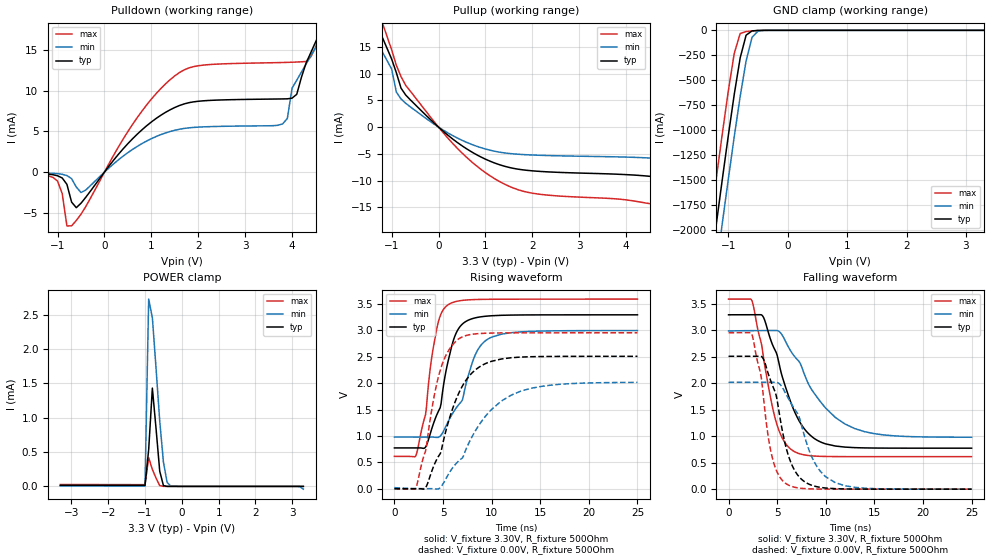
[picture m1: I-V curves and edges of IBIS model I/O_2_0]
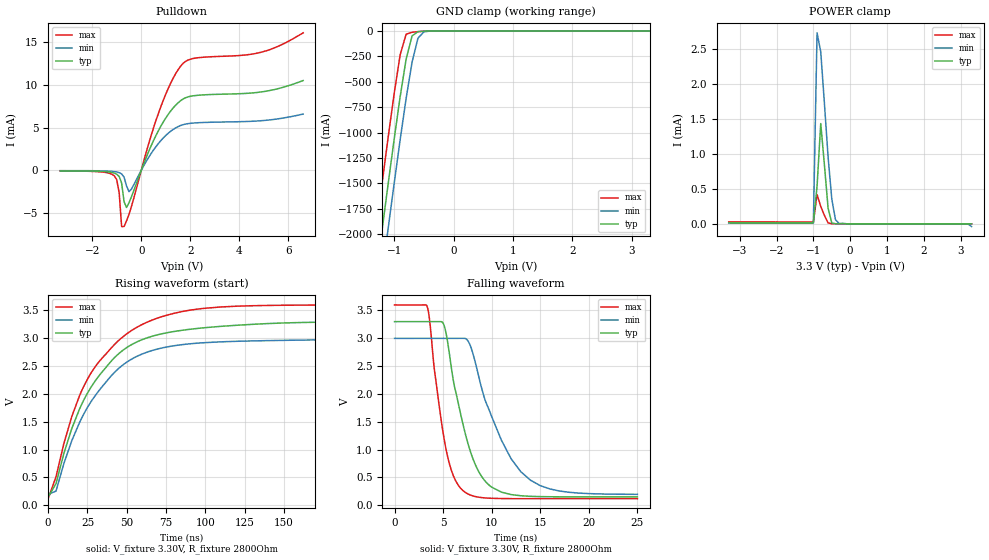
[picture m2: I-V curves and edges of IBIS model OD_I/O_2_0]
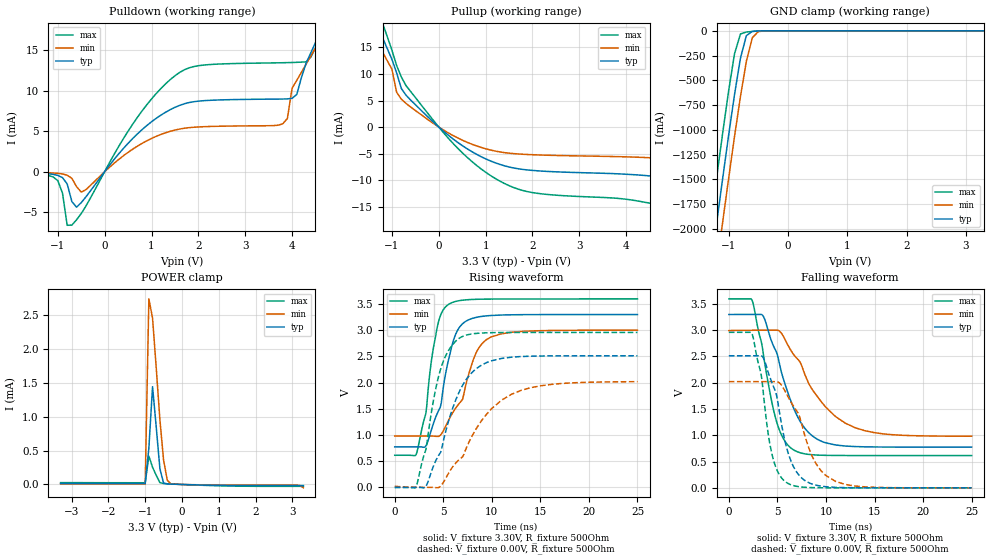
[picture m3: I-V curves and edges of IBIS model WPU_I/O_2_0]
[IBIS Ver]   3.2
[File Name]   lm3s1968_lqfp_v0p1.ibs
[File Rev]   0.1
[Date]   02/19/2010
[Source]   From silicon level SPICE simulations at Texas Instruments
[Notes]   Initial Release of IBIS model
   LM3S1968, Revision A2, 100 LQFP
[Disclaimer] Texas Instruments Confidential - Advance Product Information
   < Software License Agreement >
  Texas Instruments (TI) is supplying this software for use solely and
  exclusively on TI's Stellaris Family of microcontroller products.
  The software is owned by TI and/or its suppliers, and is protected under
  applicable copyright laws.  All rights are reserved.  Any use in violation
  of the foregoing restrictions may subject the user to criminal sanctions
  under applicable laws, as well as to civil liability for the breach of the
  terms and conditions of this license.
  THIS SOFTWARE IS PROVIDED "AS IS".  NO WARRANTIES, WHETHER EXPRESS, IMPLIED
  OR STATUTORY, INCLUDING, BUT NOT LIMITED TO, IMPLIED WARRANTIES OF
  MERCHANTABILITY AND FITNESS FOR A PARTICULAR PURPOSE APPLY TO THIS SOFTWARE.
  LMI SHALL NOT, IN ANY CIRCUMSTANCES, BE LIABLE FOR SPECIAL, INCIDENTAL, OR
  CONSEQUENTIAL DAMAGES, FOR ANY REASON WHATSOEVER.
[Copyright]   Copyright (c) 2010 Texas Instruments.  All rights reserved.
[Component]   LM3S1968 100LQFP
[Manufacturer]  Texas Instruments
[Package]
| 100-pin LQFP
| variable   typ   min   max
R_pkg   125.000m   98.000m   152.000m
L_pkg   7.745nH   6.720nH   8.770nH
C_pkg   0.745pF   0.660pF   0.830pF
[Pin]  signal_name   model_name
   1   ADC0   NC
   2   ADC1   NC
   3   VDDA   POWER
   4   GNDA   GND
   5   ADC2   NC
   6   ADC3   NC
   7   LDO   POWER
   8   VDD   POWER
   9   GND   GND
  10   PD0_IDX0   ProgBuff1
  11   PD1_PWM1   ProgBuff1
  12   PD2_U1Rx   ProgBuff1
  13   PD3_U1Tx   ProgBuff1
  14   VDD25   POWER
  15   GND   GND
  16   PG3   ProgBuff2
  17   PG2_PWM0   ProgBuff2
  18   PG1_U2Tx   ProgBuff1
  19   PG0_U2Rx   ProgBuff1
  20   VDD   POWER
  21   GND   GND
  22   PC7   ProgBuff1
  23   PC6   ProgBuff1
  24   PC5   ProgBuff1
  25   PC4_PhA0   ProgBuff1
  26   PA0_U0Rx   ProgBuff1
  27   PA1_U0Tx   ProgBuff1
  28   PA2_SSI0Clk   ProgBuff1
  29   PA3_SSI0Fss   ProgBuff1
  30   PA4_SSI0Rx   ProgBuff1
  31   PA5_SSI0Tx   ProgBuff1
  32   VDD   POWER
  33   GND   GND
  34   PA6_I2C1SCL   ProgBuff1
  35   PA7_I2C1SDA   ProgBuff1
  36   PG7_PhB1   ProgBuff2
  37   PG6_PhA1   ProgBuff2
  38   VDD25   POWER
  39   GND   GND
  40   PG5   ProgBuff2
  41   PG4_CCP3   ProgBuff2
  42   PF7   ProgBuff2
  43   PF6_CCP1   ProgBuff2
  44   VDD   POWER
  45   GND   GND
  46   PF5   ProgBuff2
  47   PF0_PhB0   ProgBuff1
  48   OSC0   NC
  49   OSC1   NC
  50   WAKE   NC
  51   HIB   NC
  52   XOSC0   NC
  53   XOSC1   NC
  54   GND   GND
  55   VBAT   POWER
  56   VDD   POWER
  57   GND   GND
  58   PF4_C0o   ProgBuff1
  59   PF3_PWM5   ProgBuff1
  60   PF2_PWM4   ProgBuff1
  61   PF1_IDX1   ProgBuff1
  62   VDD25   POWER
  63   GND   GND
  64   RST   NC
  65   CMOD0   NC
  66   PB0_CCP0   ProgBuff1
  67   PB1_CCP2   ProgBuff1
  68   VDD   POWER
  69   GND   GND
  70   PB2_I2C0SCL   ProgBuff1
  71   PB3_I2C0SDA   ProgBuff1
  72   PE0_SSI1Clk   ProgBuff1
  73   PE1_SSI1Fss   ProgBuff1
  74   PE2_SSI1Rx   ProgBuff1
  75   PE3_SSI1Tx   ProgBuff1
  76   CMOD1   NC
  77   PC3_TDO_SWO   ProgBuff1
  78   PC2_TDI   ProgBuff1
  79   PC1_TMS_SWDIO   ProgBuff1
  80   PC0_TCK_SWCLK   ProgBuff1
  81   VDD   POWER
  82   GND   GND
  83   PH3_Fault   ProgBuff2
  84   PH2   ProgBuff2
  85   PH1_PWM3   ProgBuff2
  86   PH0_PWM2   ProgBuff2
  87   GND   GND
  88   VDD25   POWER
  89   PB7_TRST   ProgBuff1
  90   PB6   ProgBuff1
  91   PB5   ProgBuff1
  92   PB4   ProgBuff1
  93   VDD   POWER
  94   GND   GND
  95   ADC7   NC
  96   ADC6   NC
  97   GNDA   GND
  98   VDDA   POWER
  99   ADC5   NC
 100   ADC4   NC
[Model Selector]   ProgBuff0
I/O_2_0   2 mA buffer without slew rate control
I/O_4_0   4 mA buffer without slew rate control
I/O_8_0   8 mA buffer without slew rate control
I/O_8S_0   8 mA buffer with slew rate control
OD_I/O_2_0   open-drain 2 mA buffer without slew rate control
OD_I/O_4_0   open-drain 4 mA buffer without slew rate control
OD_I/O_8_0   open-drain 8 mA buffer without slew rate control
OD_I/O_8S_0   open-drain 8 mA buffer with slew rate control
WPU_I/O_2_0   weak pullup 2 mA buffer without slew rate control
WPU_I/O_4_0   weak pullup 4 mA buffer without slew rate control
WPU_I/O_8_0   weak pullup 8 mA buffer without slew rate control
WPU_I/O_8S_0   weak pullup 8 mA buffer with slew rate control
WPD_I/O_2_0   weak pulldown 2 mA buffer without slew rate control
WPD_I/O_4_0   weak pulldown 4 mA buffer without slew rate control
WPD_I/O_8_0   weak pulldown 8 mA buffer without slew rate control
WPD_I/O_8S_0   weak pulldown 8 mA buffer with slew rate control
[Model Selector]   ProgBuff1
I/O_2_1   2 mA buffer without slew rate control
I/O_4_1   4 mA buffer without slew rate control
I/O_8_1   8 mA buffer without slew rate control
I/O_8S_1   8 mA buffer with slew rate control
OD_I/O_2_1   open-drain 2 mA buffer without slew rate control
OD_I/O_4_1   open-drain 4 mA buffer without slew rate control
OD_I/O_8_1   open-drain 8 mA buffer without slew rate control
OD_I/O_8S_1   open-drain 8 mA buffer with slew rate control
WPU_I/O_2_1   weak pullup 2 mA buffer without slew rate control
WPU_I/O_4_1   weak pullup 4 mA buffer without slew rate control
WPU_I/O_8_1   weak pullup 8 mA buffer without slew rate control
WPU_I/O_8S_1   weak pullup 8 mA buffer with slew rate control
WPD_I/O_2_1   weak pulldown 2 mA buffer without slew rate control
WPD_I/O_4_1   weak pulldown 4 mA buffer without slew rate control
WPD_I/O_8_1   weak pulldown 8 mA buffer without slew rate control
WPD_I/O_8S_1   weak pulldown 8 mA buffer with slew rate control
[Model Selector]   ProgBuff2
I/O_2_2   2 mA buffer without slew rate control
I/O_4_2   4 mA buffer without slew rate control
I/O_8_2   8 mA buffer without slew rate control
I/O_8S_2   8 mA buffer with slew rate control
OD_I/O_2_2   open-drain 2 mA buffer without slew rate control
OD_I/O_4_2   open-drain 4 mA buffer without slew rate control
OD_I/O_8_2   open-drain 8 mA buffer without slew rate control
OD_I/O_8S_2   open-drain 8 mA buffer with slew rate control
WPU_I/O_2_2   weak pullup 2 mA buffer without slew rate control
WPU_I/O_4_2   weak pullup 4 mA buffer without slew rate control
WPU_I/O_8_2   weak pullup 8 mA buffer without slew rate control
WPU_I/O_8S_2   weak pullup 8 mA buffer with slew rate control
WPD_I/O_2_2   weak pulldown 2 mA buffer without slew rate control
WPD_I/O_4_2   weak pulldown 4 mA buffer without slew rate control
WPD_I/O_8_2   weak pulldown 8 mA buffer without slew rate control
WPD_I/O_8S_2   weak pulldown 8 mA buffer with slew rate control
| Models and submodels in the file (48): I/O_2_0 (I/O), I/O_4_0 (I/O), I/O_8_0 (I/O), I/O_8S_0 (I/O), OD_I/O_2_0 (I/O_open_drain), OD_I/O_4_0 (I/O_open_drain), OD_I/O_8_0 (I/O_open_drain), OD_I/O_8S_0 (I/O_open_drain), WPU_I/O_2_0 (I/O), WPU_I/O_4_0 (I/O), WPU_I/O_8_0 (I/O), WPU_I/O_8S_0 (I/O), WPD_I/O_2_0 (I/O), WPD_I/O_4_0 (I/O), WPD_I/O_8_0 (I/O), WPD_I/O_8S_0 (I/O), I/O_2_1 (I/O), I/O_4_1 (I/O), I/O_8_1 (I/O), I/O_8S_1 (I/O), OD_I/O_2_1 (I/O_open_drain), OD_I/O_4_1 (I/O_open_drain), OD_I/O_8_1 (I/O_open_drain), OD_I/O_8S_1 (I/O_open_drain), WPU_I/O_2_1 (I/O), WPU_I/O_4_1 (I/O), WPU_I/O_8_1 (I/O), WPU_I/O_8S_1 (I/O), WPD_I/O_2_1 (I/O), WPD_I/O_4_1 (I/O), WPD_I/O_8_1 (I/O), WPD_I/O_8S_1 (I/O), I/O_2_2 (I/O), I/O_4_2 (I/O), I/O_8_2 (I/O), I/O_8S_2 (I/O), OD_I/O_2_2 (I/O_open_drain), OD_I/O_4_2 (I/O_open_drain), OD_I/O_8_2 (I/O_open_drain), OD_I/O_8S_2 (I/O_open_drain), WPU_I/O_2_2 (I/O), WPU_I/O_4_2 (I/O), WPU_I/O_8_2 (I/O), WPU_I/O_8S_2 (I/O), WPD_I/O_2_2 (I/O), WPD_I/O_4_2 (I/O), WPD_I/O_8_2 (I/O), WPD_I/O_8S_2 (I/O)
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[Model]   I/O_2_0
Model_type   I/O
Vinl = 1.26
Vinh = 2.04
Vmeas = 1.65
| variable   typ   min   max
C_comp   9.739pF   9.739pF   9.739pF
[Model Spec]
Vinh+   1.91   1.78   2.04
Vinh-   1.90   1.76   2.03
Vinl+   1.40   1.27   1.54
Vinl-   1.39   1.26   1.53
| variable   typ   min   max
[Temperature Range]  25   85   -40
[Voltage Range]   3.3V   3.0V   3.6V
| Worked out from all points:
|   slope of the pulldown table from 0 to 0.495 V, typ, clamps not added: 143 ohm
|   slope of the pullup table from 0 to 0.495 V, typ, clamps not added: 143 ohm
|   GND clamp passes 1 mA (typ) near -0.48 V on its own axis
|   POWER clamp passes 1 mA (typ) near -0.73 V on its own axis
|   falling waveform, V_fixture 3.30V, R_fixture 500Ohm: 20-80 % time 2.91ns typ, 4.35ns min, 1.96ns max; typ from 3.29 V to 0.774 V
|   rising waveform, V_fixture 3.30V, R_fixture 500Ohm: 20-80 % time 1.93ns typ, 2.62ns min, 1.41ns max; typ from 0.774 V to 3.3 V
|   falling waveform, V_fixture 0.00V, R_fixture 500Ohm: 20-80 % time 2ns typ, 2.73ns min, 1.46ns max; typ from 2.51 V to 0 V
|   rising waveform, V_fixture 0.00V, R_fixture 500Ohm: 20-80 % time 2.98ns typ, 4.63ns min, 1.95ns max; typ from 0.002 V to 2.51 V
[Pulldown]
|  Voltage   I(typ)   I(min)   I(max)
-3.3V     -64.15uA   -36.41uA   -91.13uA
-1.1V     -318.3uA   -146.9uA   -641.8uA
-700mV    -3.678mA   -803.7uA   -6.582mA
-500mV    -3.814mA   -2.5mA     -5.165mA
600mV     4.09mA     2.783mA    5.852mA
1.5V      7.921mA    5.13mA     11.8mA
3.8V      8.971mA    5.912mA    13.44mA
4.1V      9.534mA    11.26mA    13.49mA
4.6V      17.2mA     16.24mA    17.2mA
4.8V      19.76mA    18.22mA    20.43mA
6.5V      43.78mA    32.33mA    51.9mA
6.6V      45.47mA    7.61mA     54.43mA
[Pullup]
|  Voltage   I(typ)   I(min)   I(max)
-3.3V     58.76mA    44.69mA    74.9mA
-1.5V     22.87mA    18.92mA    27.05mA
-1.3V     18.86mA    15.72mA    22.09mA
-1.2V     16.83mA    14.11mA    19.57mA
-1V       12.74mA    10.89mA    14.48mA
-900mV    10.19mA    6.572mA    11.58mA
-600mV    5.094mA    3.782mA    6.706mA
500mV     -3.489mA   -2.46mA    -4.836mA
1.5V      -7.533mA   -4.924mA   -11.05mA
5V        -9.793mA   -6.102mA   -15.25mA
5.9V      -11.98mA   -7.296mA   -18.76mA
6.6V      -15.07mA   -8.994mA   -23.96mA
[GND Clamp]
|  Voltage   I(typ)   I(min)   I(max)
-3.3V     -11.72A    -12.12A    -11.3A
-1.4V     -2.845A    -3.285A    -2.387A
-1.3V     -2.39A     -2.831A    -1.93A
-1.2V     -1.938A    -2.38A     -1.478A
-1.1V     -1.494A    -1.934A    -1.036A
-1V       -1.059A    -1.496A    -610.6mA
-900mV    -645mA     -1.069A    -232.9mA
-800mV    -277.1mA   -664.4mA   -31.59mA
-700mV    -48.56mA   -306.6mA   -12.09mA
-600mV    -5.558mA   -70.2mA    -6.272mA
-500mV    -1.167mA   -7.88mA    -2.167mA
3.3V      2.282nA    3.101uA    451.3pA
[POWER Clamp]
|  Voltage   I(typ)   I(min)   I(max)
-3.3V     15.18uA    8.315uA    27.48uA
-1V       14.14uA    7.74uA     25.63uA
-900mV    536uA      2.726mA    416.7uA
-800mV    1.43mA     2.454mA    247.6uA
-700mV    840.7uA    1.719mA    119.9uA
-600mV    221.2uA    951.5uA    11.58uA
-500mV    12.35uA    355.6uA    955.3nA
-400mV    305.2nA    58.59uA    44.3nA
-300mV    9.515nA    3.101uA    1.472nA
3.1V      1.302nA    -112.7nA   143.5pA
3.2V      1.207nA    -2.287uA   131.7pA
3.3V      -104.8pA   -40.34uA   119.2pA
[Ramp]
| variable   typ   min   max
dV/dt_f   1.51/2.91n   1.20/4.35n   1.79/1.96n
dV/dt_r   1.50/2.98n   1.20/4.63n   1.77/1.95n
R_load = 500Ohm
[Falling Waveform]
V_fixture = 3.30V
V_fixture_min = 3.00V
V_fixture_max = 3.60V
R_fixture = 500Ohm
|   Time   V(typ)   V(min)   V(max)
0s        3.294V     2.989V     3.591V
2.4ns     3.295V     2.995V     3.563V
3.5ns     3.274V     2.996V     2.613V
4.8ns     2.619V     2.997V     1.334V
5.6ns     2.08V      2.885V     940.6mV
6.6ns     1.547V     2.554V     729.4mV
8.9ns     947.9mV    1.79V      624.9mV
11ns      814.5mV    1.352V     615.6mV
13ns      784.5mV    1.143V     614.4mV
25ns      774.3mV    980.8mV    614.1mV
[Rising Waveform]
V_fixture = 3.30V
V_fixture_min = 3.00V
V_fixture_max = 3.60V
R_fixture = 500Ohm
|   Time   V(typ)   V(min)   V(max)
0s        774.3mV    980mV      614.1mV
2.2ns     774.3mV    980mV      626.1mV
3.2ns     789.7mV    979.9mV    1.403V
3.7ns     1.052V     980mV      2.304V
4.4ns     1.419V     972.8mV    3.071V
5.6ns     2.479V     1.3V       3.495V
6.9ns     3.104V     1.656V     3.567V
8.3ns     3.238V     2.531V     3.585V
9.9ns     3.277V     2.865V     3.59V
25ns      3.296V     2.998V     3.594V
[Falling Waveform]
V_fixture = 0.00V
V_fixture_min = 0.00V
V_fixture_max = 0.00V
R_fixture = 500Ohm
|   Time   V(typ)   V(min)   V(max)
0s        2.51V      2.018V     2.956V
2.4ns     2.51V      2.018V     2.925V
3.3ns     2.51V      2.018V     2.184V
4.4ns     2.016V     2.018V     673.7mV
4.9ns     1.771V     2.018V     363mV
6ns       729.1mV    1.765V     94.24mV
7.7ns     157.2mV    1.076V     12.64mV
9.1ns     45.95mV    426.3mV    2.652mV
11ns      9.196mV    121.6mV    418.4uV
25ns      27.86uV    63.94uV    19.33uV
[Rising Waveform]
V_fixture = 0.00V
V_fixture_min = 0.00V
V_fixture_max = 0.00V
R_fixture = 500Ohm
|   Time   V(typ)   V(min)   V(max)
0s        2.208mV    22.16mV    122.2uV
2.2ns     370.3uV    5.825mV    15.25mV
3.2ns     18.81mV    3.22mV     714.1mV
4ns       412mV      1.785mV    1.668V
4.7ns     662mV      19.49mV    2.238V
5.5ns     1.235V     257.7mV    2.598V
6.7ns     1.843V     541.5mV    2.851V
8.7ns     2.303V     1.208V     2.94V
12ns      2.483V     1.774V     2.954V
25ns      2.51V      2.016V     2.955V
[Model]   OD_I/O_2_0
Model_type   I/O_open_drain
Polarity   Inverting
Vinl = 1.26
Vinh = 2.04
Vmeas = 1.65
Rref = 2800
Vref = 3.3
| variable   typ   min   max
C_comp   9.739pF   9.739pF   9.739pF
[Model Spec]
Vinh+   1.91   1.78   2.04
Vinh-   1.90   1.76   2.03
Vinl+   1.40   1.27   1.54
Vinl-   1.39   1.26   1.53
| variable   typ   min   max
[Temperature Range]  25   85   -40
[Voltage Range]   3.3V   3.0V   3.6V
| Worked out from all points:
|   slope of the pulldown table from 0 to 0.495 V, typ, clamps not added: 143 ohm
|   GND clamp passes 1 mA (typ) near -0.48 V on its own axis
|   POWER clamp passes 1 mA (typ) near -0.73 V on its own axis
|   falling waveform, V_fixture 3.30V, R_fixture 2800Ohm: 20-80 % time 2.51ns typ, 3.84ns min, 1.7ns max; typ from 3.3 V to 0.149 V
|   rising waveform, V_fixture 3.30V, R_fixture 2800Ohm: 20-80 % time 34.2ns typ, 33.9ns min, 35.2ns max; typ from 0.149 V to 3.3 V
[Pulldown]
|  Voltage   I(typ)   I(min)   I(max)
-3.3V     -64.15uA   -36.41uA   -91.13uA
-1.1V     -318.3uA   -146.9uA   -641.8uA
-900mV    -721.3uA   -265.2uA   -2.635mA
-800mV    -1.498mA   -417.6uA   -6.598mA
-700mV    -3.678mA   -803.7uA   -6.582mA
-600mV    -4.358mA   -1.83mA    -5.933mA
-500mV    -3.814mA   -2.5mA     -5.165mA
700mV     4.654mA    3.152mA    6.687mA
1.2V      6.961mA    4.59mA     10.23mA
1.7V      8.361mA    5.354mA    12.53mA
4.9V      9.201mA    5.826mA    13.87mA
6.6V      10.54mA    6.604mA    16.13mA
[GND Clamp]
|  Voltage   I(typ)   I(min)   I(max)
-3.3V     -11.72A    -12.12A    -11.3A
-1.4V     -2.845A    -3.285A    -2.387A
-1.3V     -2.39A     -2.831A    -1.93A
-1.2V     -1.938A    -2.38A     -1.478A
-1.1V     -1.494A    -1.934A    -1.036A
-1V       -1.059A    -1.496A    -610.6mA
-900mV    -645mA     -1.069A    -232.9mA
-800mV    -277.1mA   -664.4mA   -31.59mA
-700mV    -48.56mA   -306.6mA   -12.09mA
-600mV    -5.558mA   -70.2mA    -6.272mA
-500mV    -1.167mA   -7.88mA    -2.167mA
3.3V      2.282nA    3.101uA    451.3pA
[POWER Clamp]
|  Voltage   I(typ)   I(min)   I(max)
-3.3V     15.18uA    8.315uA    27.48uA
-1V       14.14uA    7.74uA     25.63uA
-900mV    536uA      2.726mA    416.7uA
-800mV    1.43mA     2.454mA    247.6uA
-700mV    840.7uA    1.719mA    119.9uA
-600mV    221.2uA    951.5uA    11.58uA
-500mV    12.35uA    355.6uA    955.3nA
-400mV    305.2nA    58.59uA    44.3nA
-300mV    9.515nA    3.101uA    1.472nA
3.1V      1.302nA    -112.7nA   143.5pA
3.2V      1.207nA    -2.287uA   131.7pA
3.3V      -104.8pA   -40.34uA   119.2pA
[Ramp]
| variable   typ   min   max
dV/dt_f   1.89/2.51n   1.68/3.84n   2.09/1.70n
dV/dt_r   1.89/34.22n   1.68/33.87n   2.09/35.22n
R_load = 2800Ohm
[Falling Waveform]
V_fixture = 3.30V
V_fixture_min = 3.00V
V_fixture_max = 3.60V
R_fixture = 2800Ohm
|   Time   V(typ)   V(min)   V(max)
0s        3.3V       2.999V     3.6V
3.4ns     3.3V       2.999V     3.551V
4.1ns     3.3V       2.999V     2.44V
5.3ns     3.098V     2.999V     1.008V
7.1ns     1.416V     2.999V     254.5mV
7.9ns     918.6mV    2.821V     176.1mV
9.3ns     438.9mV    1.903V     130.6mV
13ns      169.4mV    601.7mV    117mV
17ns      150.3mV    254.2mV    116.6mV
25ns      149mV      194.8mV    116.5mV
[Rising Waveform]
V_fixture = 3.30V
V_fixture_min = 3.00V
V_fixture_max = 3.60V
R_fixture = 2800Ohm
|   Time   V(typ)   V(min)   V(max)
0s        148.8mV    194.3mV    116.4mV
5ns       386.9mV    253.6mV    510.2mV
10ns      929.5mV    748.5mV    1.108V
15ns      1.374V     1.156V     1.59V
25ns      2.012V     1.756V     2.263V
43ns      2.673V     2.409V     2.91V
60ns      2.977V     2.719V     3.25V
82ns      3.13V      2.873V     3.46V
110ns     3.215V     2.936V     3.563V
250ns     3.298V     2.994V     3.599V
[Model]   WPU_I/O_2_0
Model_type   I/O
Vinl = 1.26
Vinh = 2.04
Vmeas = 1.65
| variable   typ   min   max
C_comp   9.739pF   9.739pF   9.739pF
[Model Spec]
Vinh+   1.91   1.78   2.04
Vinh-   1.90   1.76   2.03
Vinl+   1.40   1.27   1.54
Vinl-   1.39   1.26   1.53
| variable   typ   min   max
[Temperature Range]  25   85   -40
[Voltage Range]   3.3V   3.0V   3.6V
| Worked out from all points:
|   slope of the pulldown table from 0 to 0.495 V, typ, clamps not added: 143 ohm
|   slope of the pullup table from 0 to 0.495 V, typ, clamps not added: 143 ohm
|   GND clamp passes 1 mA (typ) near -0.48 V on its own axis
|   POWER clamp passes 1 mA (typ) near -0.73 V on its own axis
|   falling waveform, V_fixture 3.30V, R_fixture 500Ohm: 20-80 % time 2.91ns typ, 4.35ns min, 1.96ns max; typ from 3.29 V to 0.774 V
|   rising waveform, V_fixture 3.30V, R_fixture 500Ohm: 20-80 % time 1.93ns typ, 2.62ns min, 1.41ns max; typ from 0.774 V to 3.3 V
|   falling waveform, V_fixture 0.00V, R_fixture 500Ohm: 20-80 % time 2ns typ, 2.73ns min, 1.46ns max; typ from 2.51 V to 0 V
|   rising waveform, V_fixture 0.00V, R_fixture 500Ohm: 20-80 % time 2.98ns typ, 4.63ns min, 1.95ns max; typ from 0.002 V to 2.51 V
[Pulldown]
|  Voltage   I(typ)   I(min)   I(max)
-3.3V     -63.97uA   -36.29uA   -90.89uA
-1.1V     -317.2uA   -146.3uA   -639.6uA
-700mV    -3.674mA   -802.3uA   -6.561mA
-500mV    -3.8mA     -2.497mA   -5.141mA
600mV     4.106mA    2.793mA    5.879mA
1.5V      7.937mA    5.14mA     11.83mA
3.8V      8.962mA    5.903mA    13.43mA
4.1V      9.518mA    11.26mA    13.48mA
4.6V      17.2mA     16.24mA    17.2mA
4.8V      19.76mA    18.22mA    20.43mA
6.5V      43.78mA    32.33mA    51.9mA
6.6V      45.47mA    7.61mA     54.43mA
[Pullup]
|  Voltage   I(typ)   I(min)   I(max)
-3.3V     58.76mA    44.69mA    74.9mA
-1.5V     22.87mA    18.92mA    27.05mA
-1.3V     18.86mA    15.72mA    22.09mA
-1.2V     16.83mA    14.11mA    19.57mA
-1V       12.74mA    10.89mA    14.48mA
-900mV    10.18mA    6.552mA    11.57mA
-600mV    5.084mA    3.776mA    6.691mA
500mV     -3.481mA   -2.455mA   -4.825mA
1.5V      -7.517mA   -4.915mA   -11.03mA
5V        -9.793mA   -6.102mA   -15.25mA
5.9V      -11.98mA   -7.296mA   -18.76mA
6.6V      -15.07mA   -8.994mA   -23.96mA
[GND Clamp]
|  Voltage   I(typ)   I(min)   I(max)
-3.3V     -11.72A    -12.12A    -11.3A
-1.4V     -2.845A    -3.285A    -2.387A
-1.3V     -2.39A     -2.831A    -1.93A
-1.2V     -1.938A    -2.38A     -1.478A
-1.1V     -1.494A    -1.934A    -1.036A
-1V       -1.059A    -1.496A    -610.6mA
-900mV    -645mA     -1.069A    -232.9mA
-800mV    -277.1mA   -664.4mA   -31.6mA
-700mV    -48.56mA   -306.6mA   -12.11mA
-600mV    -5.565mA   -70.2mA    -6.295mA
-500mV    -1.181mA   -7.883mA   -2.191mA
3.3V      2.282nA    6.919uA    -6.845uA
[POWER Clamp]
|  Voltage   I(typ)   I(min)   I(max)
-3.3V     15.18uA    8.315uA    27.48uA
-1V       14.14uA    7.74uA     25.63uA
-900mV    539.2uA    2.746mA    419.4uA
-800mV    1.446mA    2.463mA    255uA
-700mV    851uA      1.726mA    135.8uA
-600mV    231.3uA    957.3uA    27.23uA
-500mV    21.69uA    361.2uA    14.14uA
-400mV    7.764uA    63.51uA    10.49uA
-300mV    5.5uA      6.919uA    7.727uA
3.1V      -16.64uA   -9.947uA   -27.43uA
3.2V      -16.65uA   -12.11uA   -27.44uA
3.3V      -16.65uA   -49.87uA   -27.45uA
[Ramp]
| variable   typ   min   max
dV/dt_f   1.51/2.91n   1.20/4.35n   1.79/1.96n
dV/dt_r   1.50/2.98n   1.20/4.63n   1.77/1.95n
R_load = 500Ohm
[Falling Waveform]
V_fixture = 3.30V
V_fixture_min = 3.00V
V_fixture_max = 3.60V
R_fixture = 500Ohm
|   Time   V(typ)   V(min)   V(max)
0s        3.294V     2.989V     3.591V
2.4ns     3.295V     2.995V     3.563V
3.5ns     3.274V     2.996V     2.613V
4.8ns     2.619V     2.997V     1.334V
5.6ns     2.08V      2.885V     940.6mV
6.6ns     1.547V     2.554V     729.4mV
8.9ns     947.9mV    1.79V      624.9mV
11ns      814.5mV    1.352V     615.6mV
13ns      784.5mV    1.143V     614.4mV
25ns      774.3mV    980.8mV    614.1mV
[Rising Waveform]
V_fixture = 3.30V
V_fixture_min = 3.00V
V_fixture_max = 3.60V
R_fixture = 500Ohm
|   Time   V(typ)   V(min)   V(max)
0s        774.3mV    980mV      614.1mV
2.2ns     774.3mV    980mV      626.1mV
3.2ns     789.7mV    979.9mV    1.403V
3.7ns     1.052V     980mV      2.304V
4.4ns     1.419V     972.8mV    3.071V
5.6ns     2.479V     1.3V       3.495V
6.9ns     3.104V     1.656V     3.567V
8.3ns     3.238V     2.531V     3.585V
9.9ns     3.277V     2.865V     3.59V
25ns      3.296V     2.998V     3.594V
[Falling Waveform]
V_fixture = 0.00V
V_fixture_min = 0.00V
V_fixture_max = 0.00V
R_fixture = 500Ohm
|   Time   V(typ)   V(min)   V(max)
0s        2.51V      2.018V     2.956V
2.4ns     2.51V      2.018V     2.925V
3.3ns     2.51V      2.018V     2.184V
4.4ns     2.016V     2.018V     673.7mV
4.9ns     1.771V     2.018V     363mV
6ns       729.1mV    1.765V     94.24mV
7.7ns     157.2mV    1.076V     12.64mV
9.1ns     45.95mV    426.3mV    2.652mV
11ns      9.196mV    121.6mV    418.4uV
25ns      27.86uV    63.94uV    19.33uV
[Rising Waveform]
V_fixture = 0.00V
V_fixture_min = 0.00V
V_fixture_max = 0.00V
R_fixture = 500Ohm
|   Time   V(typ)   V(min)   V(max)
0s        2.21mV     22.16mV    122.3uV
2.2ns     370.3uV    5.826mV    15.25mV
3.2ns     18.81mV    3.22mV     714.1mV
4ns       412mV      1.785mV    1.668V
4.7ns     662mV      19.49mV    2.238V
5.5ns     1.235V     257.7mV    2.598V
6.7ns     1.843V     541.5mV    2.851V
8.7ns     2.303V     1.208V     2.94V
12ns      2.483V     1.774V     2.954V
25ns      2.51V      2.016V     2.955V
